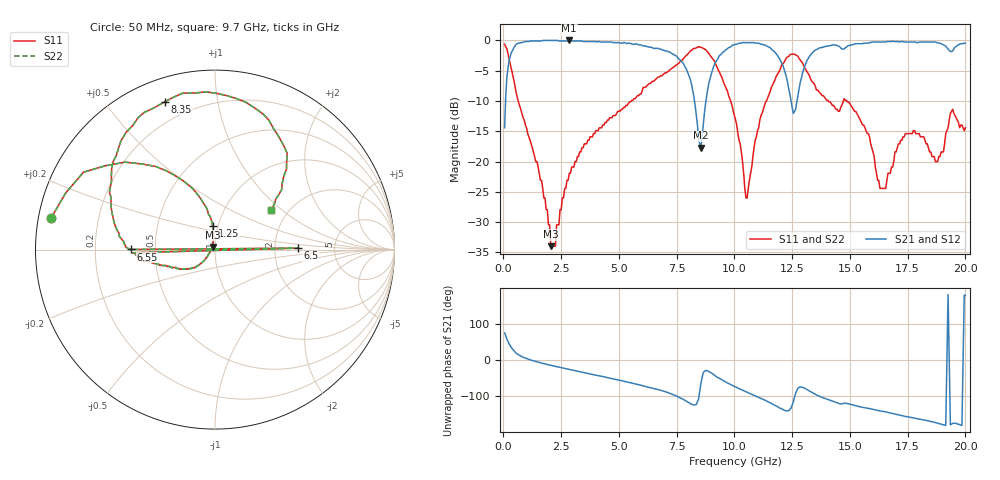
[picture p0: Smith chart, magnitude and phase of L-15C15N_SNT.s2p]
#	mhz	s	ma	r	50
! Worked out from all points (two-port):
!   400 points, 50 MHz to 20 GHz, reference 50 ohm
!   highest |S21| = 0.00 dB at 2.85 GHz (marker M1); lowest = -17.7 dB at 8.55 GHz (marker M2)
!   |S21| within 3 dB of the highest: 265.4 MHz to 7.58 GHz (7.315 GHz wide, 186 % of centre); 13.19 GHz to end of sweep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
!   lowest |S11| = -34.0 dB at 2.05 GHz (marker M3), VSWR 1.04, Z = 48.7 + j1.47 ohm
!   |S11| at or under -10 dB: 639.2 MHz to 5.531 GHz (4.892 GHz wide, 159 % of centre); 9.834 GHz to 11.38 GHz (1.547 GHz wide, 14.6 % of centre); 14.87 GHz to end of sweep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
!   |S22| runs from -34.0 to -0.6 dB; largest |S21 - S12| = 0
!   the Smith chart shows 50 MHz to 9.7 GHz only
!   S11 on the Smith chart (normalised r, x): 50 MHz: 0.04, +0.10; 1.25 GHz: 0.94, +0.25; 6.5 GHz: 2.70, +0.06; 6.55 GHz: 0.36, +0.00; 8.35 GHz: 0.11, +0.71; 9.7 GHz: 1.63, +0.84
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50  0.93 169.1  0.19 74.6  0.19 74.6  0.93 169.1
1250  0.13 95.5  0.99 -1.4  0.99 -1.4  0.13 95.5
2050  0.02 131.0  1 -14.7  1 -14.7  0.02 131.0
2850  0.08 -134.9  1 -26.1  1 -26.1  0.08 -134.9
3400  0.13 -136.6  0.99 -33.6  0.99 -33.6  0.13 -136.6
6500  0.46 1.0  0.86 -78.4  0.86 -78.4  0.46 1.0
6550  0.47 179.9  0.86 -79.2  0.86 -79.2  0.47 179.9
6700  0.5 178.0  0.86 -81.3  0.86 -81.3  0.5 178.0
8350  0.87 108.7  0.24 -122.2  0.24 -122.2  0.87 108.7
8550  0.88 93.0  0.13 -64.0  0.13 -64.0  0.88 93.0
9700  0.38 35.5  0.86 -63.1  0.86 -63.1  0.38 35.5
10050  0.22 30.0  0.93 -73.7  0.93 -73.7  0.22 30.0
13350  0.46 11.4  0.78 -89.2  0.78 -89.2  0.46 11.4
16700  0.08 95.2  0.98 -144.9  0.98 -144.9  0.08 95.2
19150  0.17 16.0  0.9 -179.8  0.9 -179.8  0.17 16.0
19200  0.18 6.6  0.87 0.0  0.87 0.0  0.18 6.6
19250  0.19 -2.8  0.85 179.7  0.85 179.7  0.19 -2.8
19300  0.22 -9.0  0.83 0.7  0.83 0.7  0.22 -9.0
19350  0.25 -15.1  0.81 -178.2  0.81 -178.2  0.25 -15.1
19850  0.2 -55.7  0.94 -179.6  0.94 -179.6  0.2 -55.7
19900  0.19 -54.2  0.94 -0.8  0.94 -0.8  0.19 -54.2
20000  0.19 -51.0  0.95 177.2  0.95 177.2  0.19 -51.0
